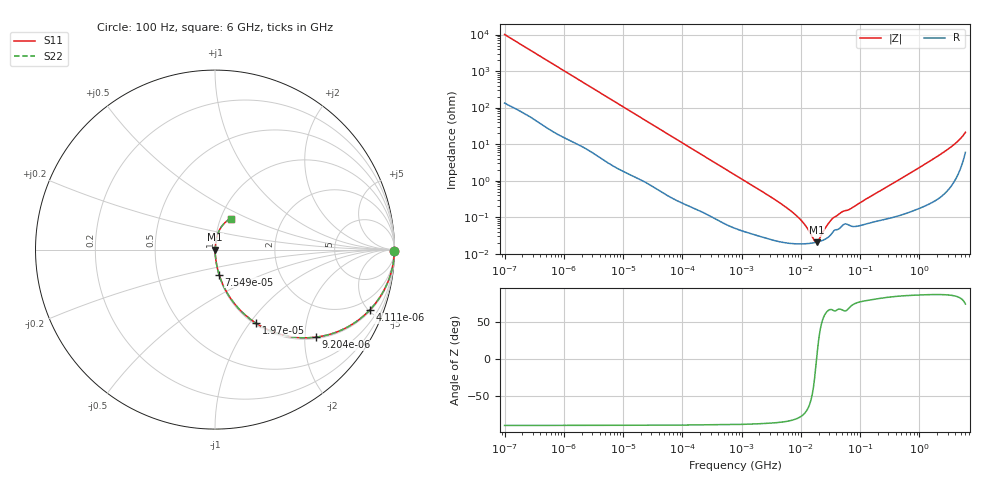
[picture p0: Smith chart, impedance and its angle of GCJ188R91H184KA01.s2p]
!Murata Part Number: GCJ188R91H184KA01
!These Parameters are Measured in Series Mode Connection
!Data Generated on Mar 13, 2026
!  o--ll--o
!Port1  Port2
!  o------o
!Operation Temp=25[degC], DC Bias Voltage=0[V]
!Freq. Start=100[Hz] Stop=6[GHz] 401[Steps]
# Hz S RI R 50
!Freq.(Hz) S11(Real) S11(Imag) S21(Real) S21(Imag) S12(Real) S12(Imag) S22(Real) S22(Imag)
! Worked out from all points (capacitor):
!   401 points, 100 Hz to 6 GHz, reference 50 ohm
!   read as one part in series: C = 158 nF near 109 Hz
!   lowest |Z| = 20.6 mohm at 18.61 MHz (marker M1)
!   series resonance near 18.48 MHz, so ESL is about 470 pH
!   S11 on the Smith chart (normalised r, x): 100 Hz: open; 4.111 kHz: 1.08, -5.06; 9.204 kHz: 1.04, -2.28; 19.7 kHz: 1.02, -1.07; 75.5 kHz: 1.01, -0.28; 6 GHz: 1.12, +0.40
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100  0.9998 -0.00996  0.000231 0.00996  0.000231 0.00996  0.9998 -0.00996
600  0.9957 -0.0584  0.00425 0.0584  0.00425 0.0584  0.9957 -0.0584
2008  0.9606 -0.1863  0.0394 0.1863  0.0394 0.1863  0.9606 -0.1863
4111  0.8609 -0.3378  0.1391 0.3378  0.1391 0.3378  0.8609 -0.3378
9204  0.5636 -0.4876  0.4364 0.4876  0.4364 0.4876  0.5636 -0.4876
19704  0.2281 -0.4098  0.7719 0.4098  0.7719 0.4098  0.2281 -0.4098
40335  0.0699 -0.2449  0.9301 0.2449  0.9301 0.2449  0.0699 -0.2449
75495  0.0227 -0.1388  0.9773 0.1388  0.9773 0.1388  0.0227 -0.1388
193316  0.00465 -0.056  0.9953 0.056  0.9953 0.056  0.00465 -0.056
774597  0.000698 -0.0143  0.9993 0.0143  0.9993 0.0143  0.000698 -0.0143
3394479  0.000244 -0.00325  0.9998 0.00325  0.9998 0.00325  0.000244 -0.00325
6948629  0.000191 -0.00142  0.9998 0.00142  0.9998 0.00142  0.000191 -0.00142
1.087309e7  0.000186 -0.000695  0.9998 0.000695  0.9998 0.000695  0.000186 -0.000695
1.555665e7  0.000195 -0.000217  0.9998 0.000217  0.9998 0.000217  0.000195 -0.000217
1.701401e7  0.0002 -0.000103  0.9998 0.000103  0.9998 0.000103  0.0002 -0.000103
1.86079e7  0.000206 9.1e-06  0.9998 -9.1e-06  0.9998 -9.1e-06  0.000206 9.1e-06
2.035112e7  0.000214 0.000122  0.9998 -0.000122  0.9998 -0.000122  0.000214 0.000122
2.911731e7  0.000282 0.000603  0.9997 -0.000603  0.9997 -0.000603  0.000282 0.000603
3.64232e7  0.00043 0.000893  0.9996 -0.000893  0.9996 -0.000893  0.00043 0.000893
3.124326e8  0.00098 0.0073  0.999 -0.0073  0.999 -0.0073  0.00098 0.0073
2.562649e9  0.00759 0.0588  0.9924 -0.0588  0.9924 -0.0588  0.00759 0.0588
6e9  0.089 0.1732  0.911 -0.1732  0.911 -0.1732  0.089 0.1732
